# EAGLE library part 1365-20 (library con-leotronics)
DUAL ROW STRAIGHT HEADER 1364 SERIES. 1.27mm x 1.27mm. Without Fixing Post. SMT Source: http://www.leotronics.co.uk/Conexcon/Data%20Sheets/sec.%20A/1364ing.pdf
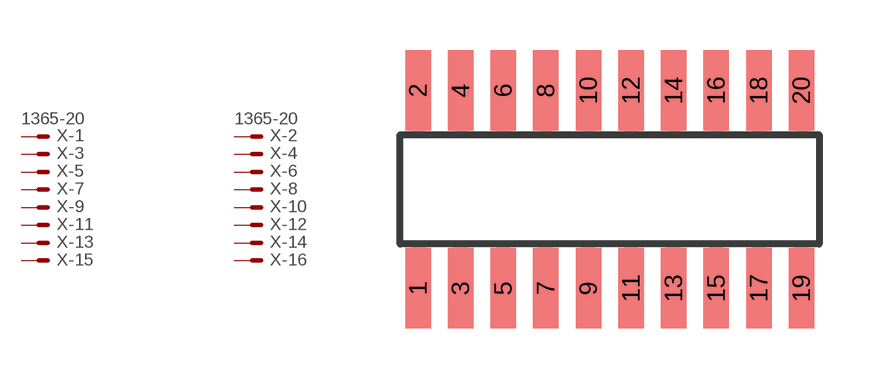
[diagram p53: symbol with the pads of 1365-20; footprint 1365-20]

Designator prefix X; gates -1=MVAL -2=MVAL -3=M -4=M -5=M -6=M -7=M -8=M -9=M -10=M -11=M -12=M -13=M -14=M -15=M -16=M -17=M -18=M -19=M -20=M

## 1365-20 (OC_FARNELL: unknown; OC_NEWARK: unknown)  [1365-20]
1  -1:S  pas
2  -2:S  pas
3  -3:S  pas
4  -4:S  pas
5  -5:S  pas
6  -6:S  pas
7  -7:S  pas
8  -8:S  pas
9  -9:S  pas
10  -10:S  pas
11  -11:S  pas
12  -12:S  pas
13  -13:S  pas
14  -14:S  pas
15  -15:S  pas
16  -16:S  pas
17  -17:S  pas
18  -18:S  pas
19  -19:S  pas
20  -20:S  pas

## Footprint 1365-20 (pad centres in mm)
DUAL ROW STRAIGHT HEADER 1364 SERIES. 1.27mm x 1.27mm. Without Fixing Post. SMT Source: http://www.leotronics.co.uk/Conexcon/Data%20Sheets/sec.%20A/1364ing.pdf
smd 0.76 x 2.4: 1 -5.715,-2.95; 2 -5.715,2.95; 3 -4.445,-2.95; 4 -4.445,2.95; 5 -3.175,-2.95; 6 -3.175,2.95; 7 -1.905,-2.95; 8 -1.905,2.95; 9 -0.635,-2.95; 10 -0.635,2.95; 11 0.635,-2.95; 12 0.635,2.95; 13 1.905,-2.95; 14 1.905,2.95; 15 3.175,-2.95; 16 3.175,2.95; 17 4.445,-2.95; 18 4.445,2.95; 19 5.715,-2.95; 20 5.715,2.95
